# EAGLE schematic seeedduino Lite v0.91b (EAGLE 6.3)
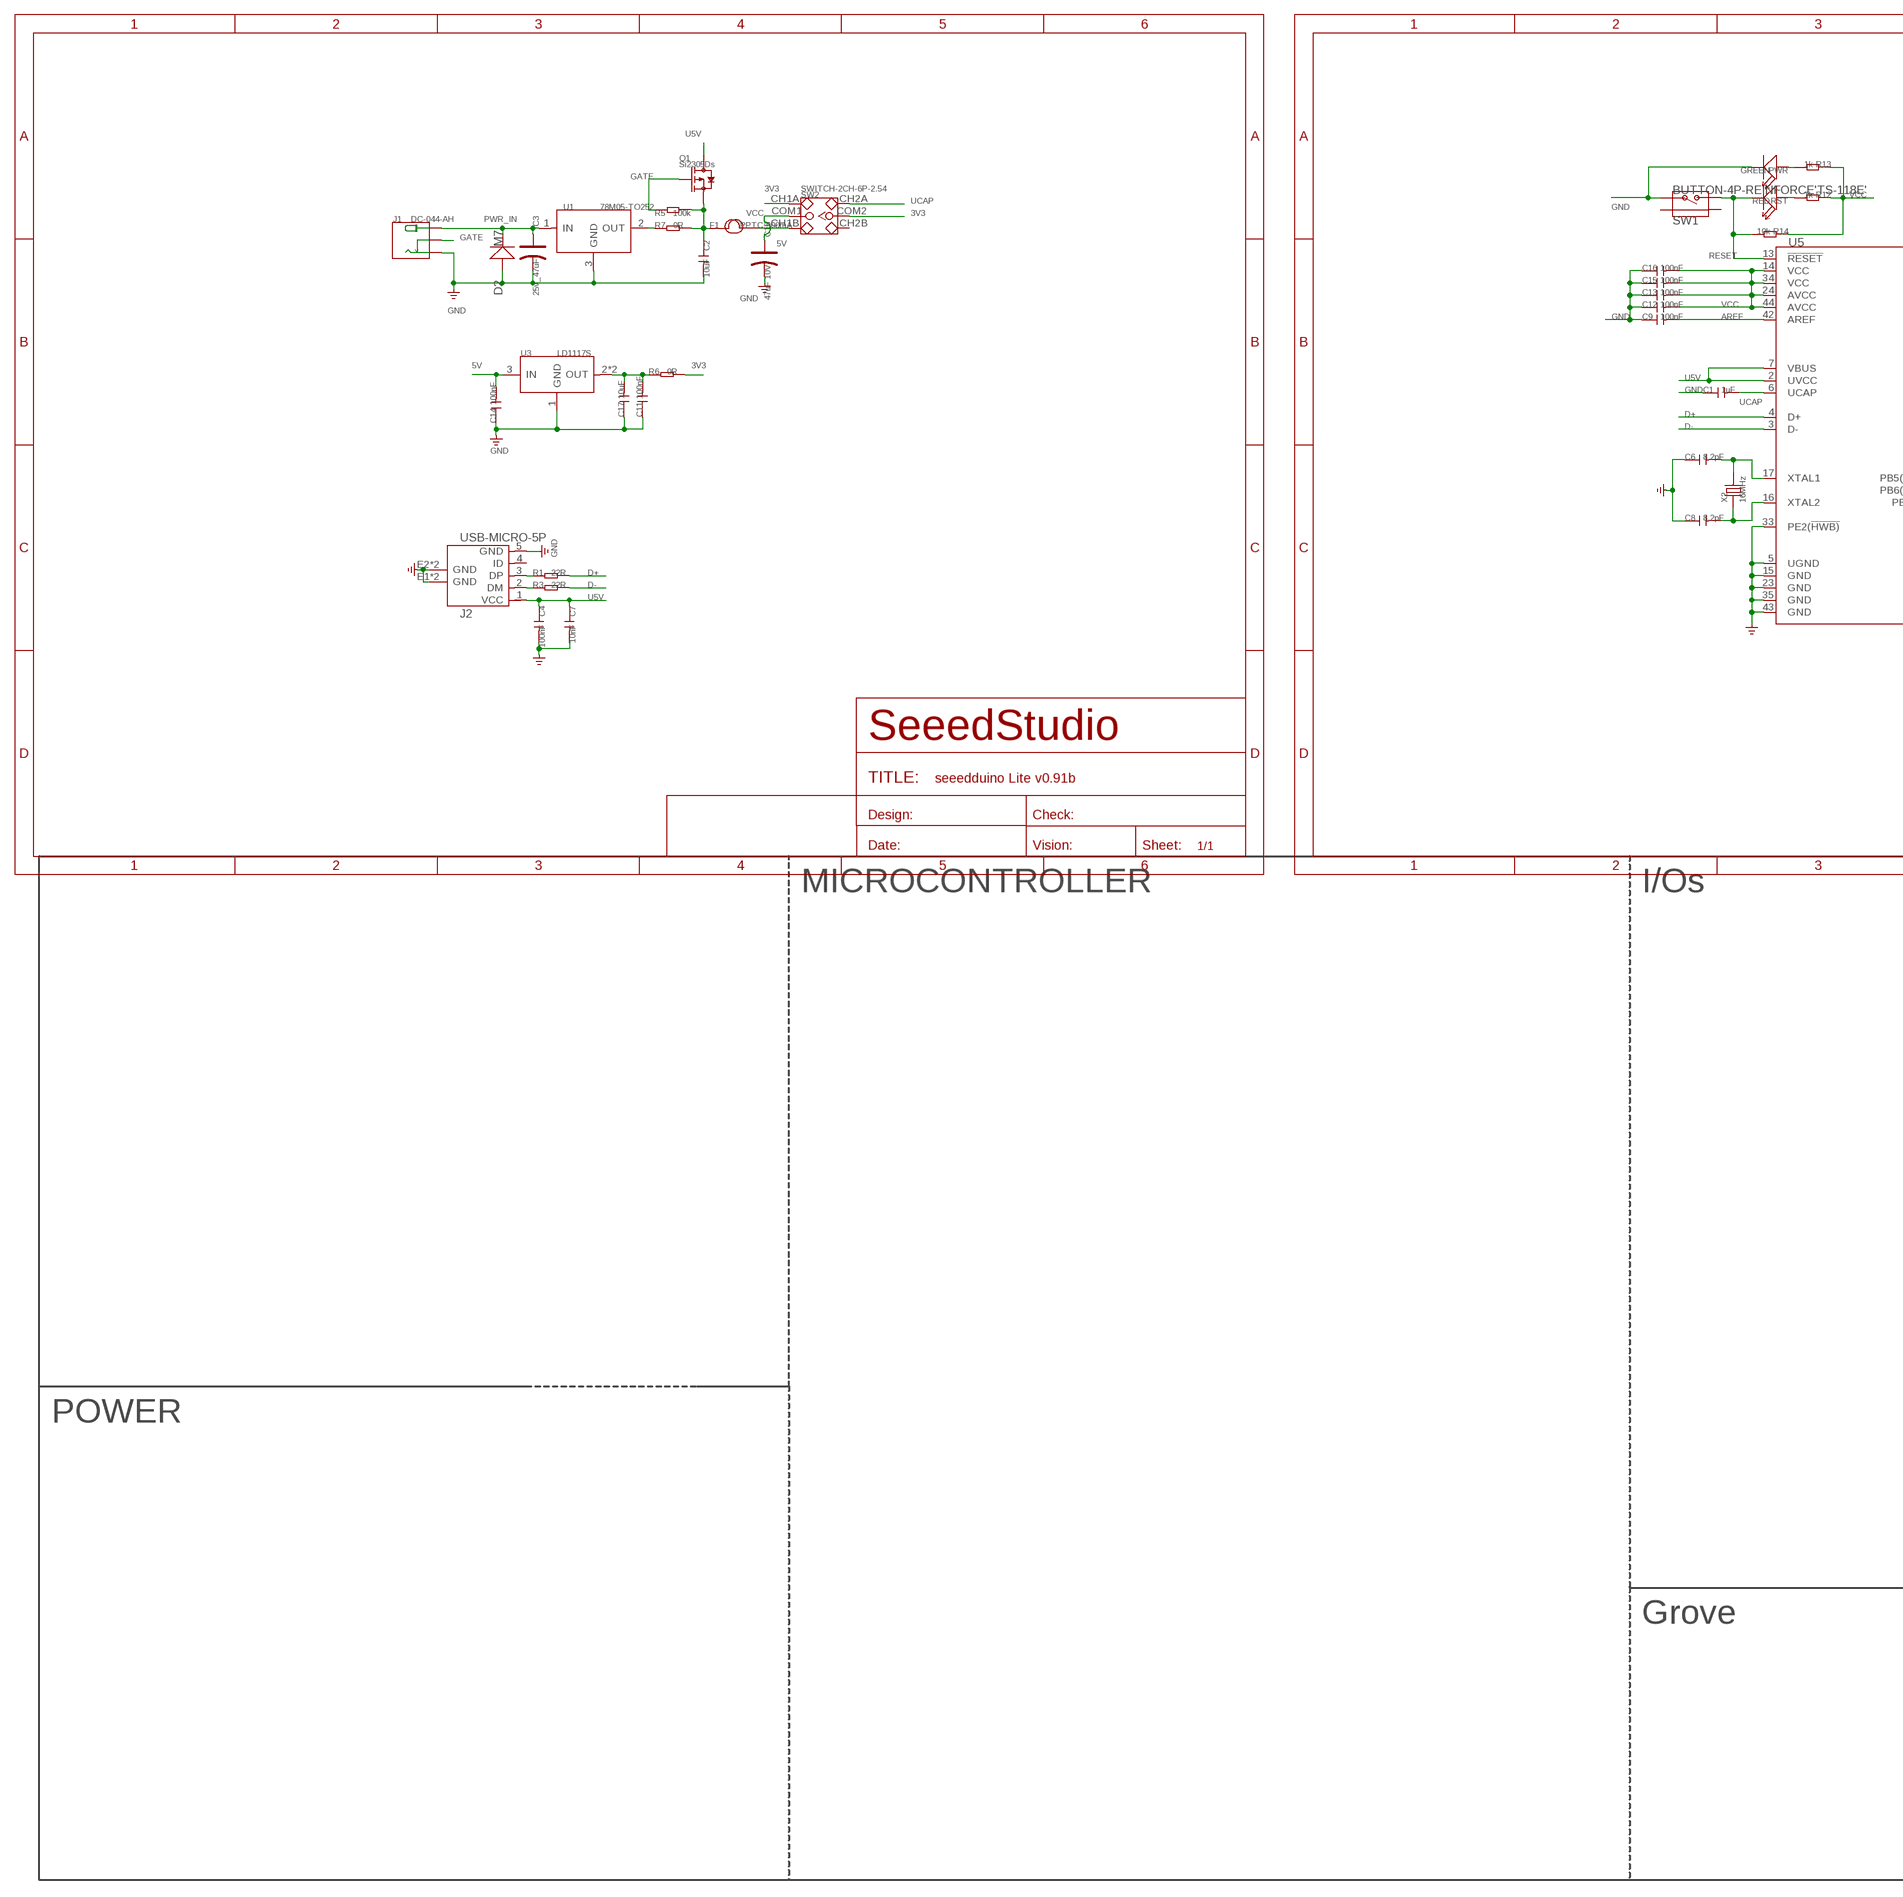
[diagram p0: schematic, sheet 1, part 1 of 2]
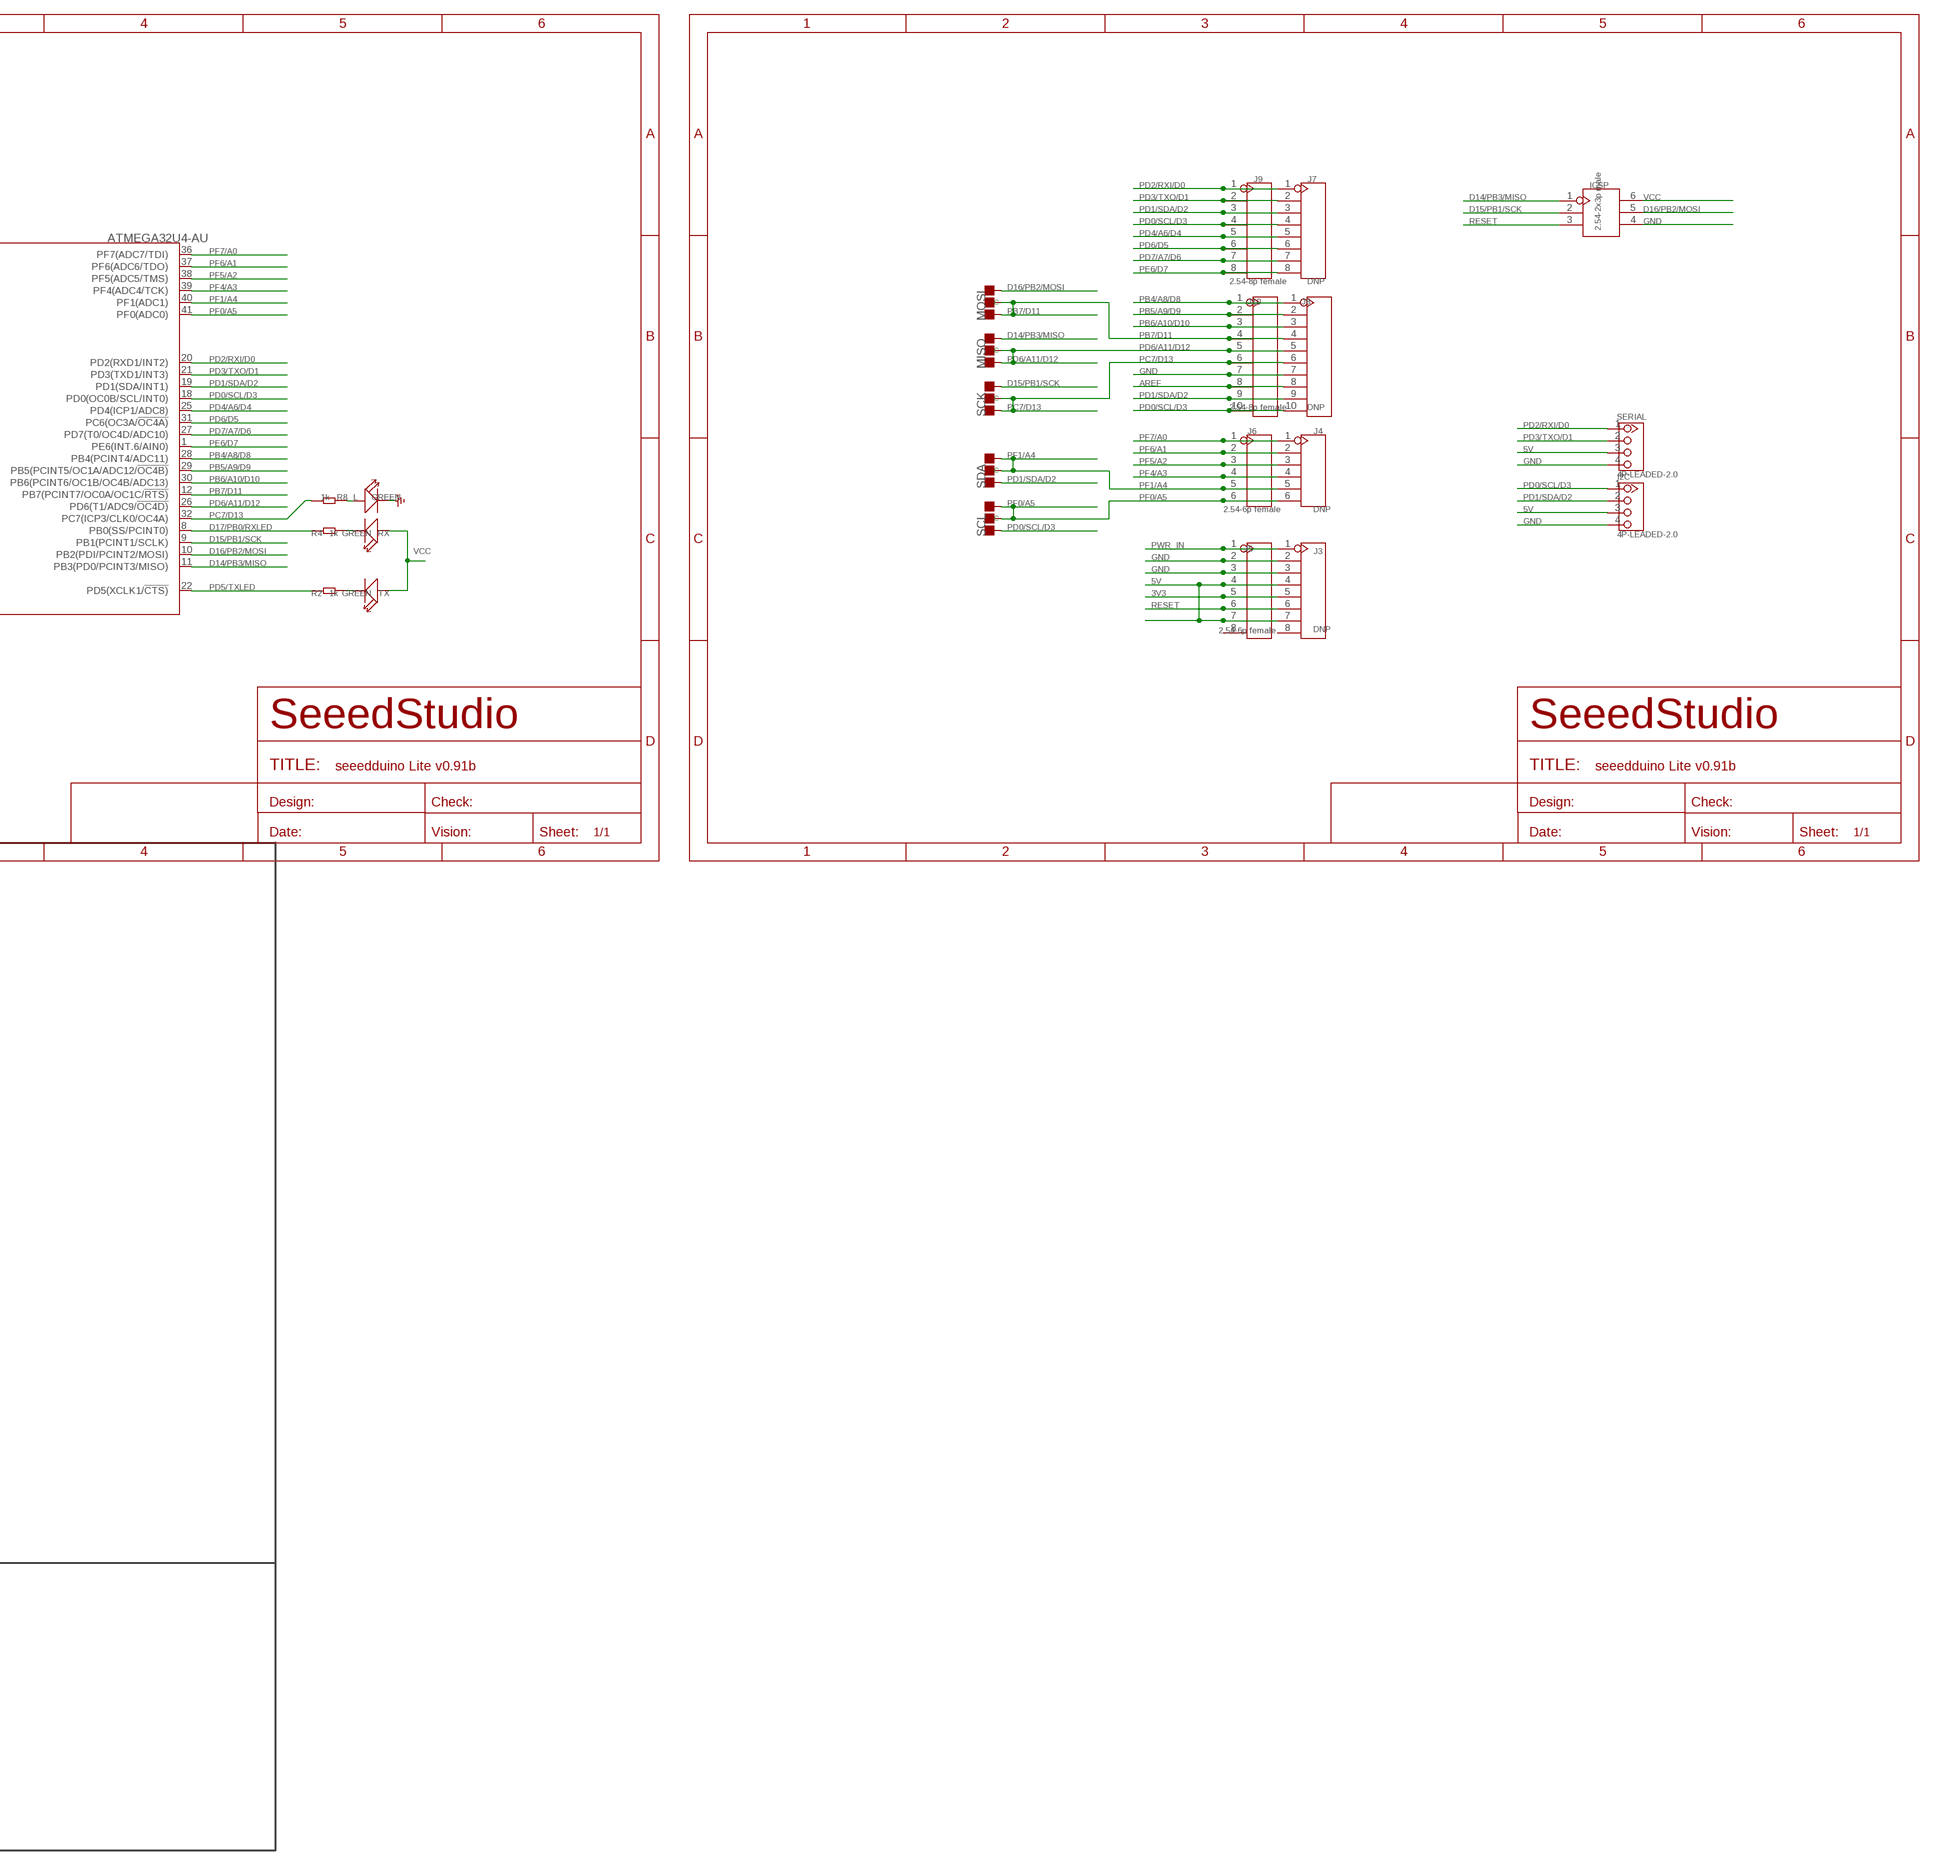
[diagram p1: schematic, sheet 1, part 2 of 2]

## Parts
C1  1uF  C-0805  [C0805]
C2  10uF  C-0805  [C0805]
C3  25v_47uF  CAP-ELECTRO-C  [ELECTRO-SMD-C-6MM]
C4  100nF  C-0603  [C0603]
C6  8.2pF  C-0603  [C0603]
C7  10nF  C-0603  [C0603]
C8  8.2pF  C-0603  [C0603]
C9  100nF  C-0603  [C0603]
C10  47uF 10V  CAP-AVX-B  [AVX-B]
C11  100nF  C-0603  [C0603]
C12  100nF  C-0603  [C0603]
C13  100nF  C-0603  [C0603]
C14  100nF  C-0603  [C0603]
C15  100nF  C-0603  [C0603]
C16  100nF  C-0603  [C0603]
C17  10uF  C-0805  [C0805]
D2  M7  D'SMA'  [D2010]
F1  PPTC-500mA  FUSE'1206'  [F1206]
I2C  4P-LEADED-2.0  TWIG-2.0-LEADED  [4P-LEADED-2.0]
ICSP  2.54-2x3p male  HEADER-2X3P-2.54  [2X3P-2.54]
J1  DC-044-AH  DC-044  [DC-404]
J2  USB-MICRO-5P  [MICRO-USB-5P]
J3  DNP  HEADER-8P-65/35MIL  [8P-2.54-65/35MIL]
J4  DNP  HEADER-6P-65/35MIL  [6P-2.54-65/35MIL]
J5  2.54-6p female  HEADER-8P-65/35MIL  [8P-2.54-65/35MIL]
J6  2.54-6p female  HEADER-6P-65/35MIL  [6P-2.54-65/35MIL]
J7  DNP  HEADER-8P-65/35MIL  [8P-2.54-65/35MIL]
J8  DNP  HEADER-10P-2.54  [10P-2.54]
J9  2.54-8p female  HEADER-8P-65/35MIL  [8P-2.54-65/35MIL]
J10  2.54-8p female  HEADER-10P-2.54  [10P-2.54]
L  GREEN  LED'0603'  [LED-0603]
MISO  DNP  PAD-JUMPER-3P-40*40  [3P-SMD-4.1X1.5]
MOSI  DNP  PAD-JUMPER-3P-40*40  [3P-SMD-4.1X1.5]
PWR  GREEN  LED'0603'  [LED-0603]
Q1  Si2305Ds  MOSFET-P'SI2323CDS/SI2305DS<BR>'  [SOT23]
R1  22R  R-0603  [R0603]
R2  1k  R-0603  [R0603]
R3  22R  R-0603  [R0603]
R4  1k  R-0603  [R0603]
R5  100k  R-0603  [R0603]
R6  0R  R-0603  [R0603]
R7  0R  R-0603  [R0603]
R8  1k  R-0603  [R0603]
R12  1k  R-0603  [R0603]
R13  1k  R-0603  [R0603]
R14  10k  R-0603  [R0603]
RST  RED  LED'0603'  [LED-0603]
RX  GREEN  LED'0603'  [LED-0603]
SCK  DNP  PAD-JUMPER-3P-40*40  [3P-SMD-4.1X1.5]
SCL  DNP  PAD-JUMPER-3P-40*40  [3P-SMD-4.1X1.5]
SDA  DNP  PAD-JUMPER-3P-40*40  [3P-SMD-4.1X1.5]
SERIAL  4P-LEADED-2.0  TWIG-2.0-LEADED  [4P-LEADED-2.0]
SW1  BUTTON-4P-REINFORCE'TS-118E'  [4P-SMD-7X3.5X3.5H]
SW2  SWITCH-2CH-6P-2.54  SWITCH-2CH-6P'MS-22D18'  [6P-2CH-2.5-9.1X3.5X3.2H]
TX  GREEN  LED'0603'  [LED-0603]
U1  78M05-TO252  [TO252]
U3  LD1117S  [SOT-223]
U5  ATMEGA32U4-AU  [TQFP44]
X2  16MHz  CRYSTAL'5032'  [2P-SMD-5X3.2]

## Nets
3V3: J3.5 J5.5 R6.2 SW2.CH1A SW2.COM2
5V [none3]: C14.2 F1.2 I2C.3 J3.4 J3.7 J5.4 J5.7 SERIAL.3 SW2.CH1B U3.3(IN)
AREF: C9.2 J8.8 J10.8 U5.42(AREF)
D14/PB3/MISO: ICSP.1 MISO.00(L) U5.11(PB3(PD0/PCINT3/MISO))
D15/PB1/SCK: ICSP.2 SCK.00(L) U5.9(PB1(PCINT1/SCLK))
D16/PB2/MOSI: ICSP.5 MOSI.00(L) U5.10(PB2(PDI/PCINT2/MOSI))
D17/PB0/RXLED: R4.1 U5.8(PB0(SS/PCINT0))
D+: R1.2 U5.4(D+)
D-: R3.2 U5.3(D-)
GATE: J1.CDN Q1.1(G) R5.1
GND [none1]: C1.1 C2.2 C3.- C4.2 C6.1 C7.2 C8.1 C9.1 C10.- C11.1 C12.1 C13.1 C14.1 C15.1 C16.1 C17.1 D2.+ I2C.4 ICSP.4 J1.- J2.5(GND) J2.E1(GND) J2.E2(GND) J2.P1(GND) J2.P2(GND) J3.2 J3.3 J5.2 J5.3 J8.7 J10.7 L.- PWR.- SERIAL.4 SW1.1 U1.3(GND) U3.1(GND) U5.5(UGND) U5.15(GND) U5.23(GND) U5.33(PE2(!HWB)) U5.35(GND) U5.43(GND)
N$1: C6.2 U5.17(XTAL1) X2.2
N$2: C8.2 U5.16(XTAL2) X2.1
N$3: C11.2 C17.2 R6.1 U3.2(OUT) U3.TER(OUT)
N$4: L.+ R8.1
N$5: R2.2 TX.-
N$6: J2.2(DM) R3.1
N$7: R4.2 RX.-
N$8: J2.3(DP) R1.1
N$9: C2.1 F1.1 Q1.2(S) R5.2 R7.2
N$10: PWR.+ R13.2
N$11: R7.1 U1.2(OUT)
N$17: R12.2 RST.+
PB4/A8/D8: J8.1 J10.1 U5.28(PB4(PCINT4/ADC11))
PB5/A9/D9: J8.2 J10.2 U5.29(PB5(PCINT5/OC1A/ADC12/!OC4B))
PB6/A10/D10: J8.3 J10.3 U5.30(PB6(PCINT6/OC1B/OC4B/ADC13))
PB7/D11: J8.4 J10.4 MOSI.11(R) MOSI.MM(C) U5.12(PB7(PCINT7/OC0A/OC1C/!RTS))
PC7/D13: J8.6 J10.6 R8.2 SCK.11(R) SCK.MM(C) U5.32(PC7(ICP3/CLK0/OC4A))
PD0/SCL/D3: I2C.1 J7.4 J8.10 J9.4 J10.10 SCL.11(R) U5.18(PD0(OC0B/SCL/INT0))
PD1/SDA/D2: I2C.2 J7.3 J8.9 J9.3 J10.9 SDA.11(R) U5.19(PD1(SDA/INT1))
PD2/RXI/D0: J7.1 J9.1 SERIAL.1 U5.20(PD2(RXD1/INT2))
PD3/TXO/D1: J7.2 J9.2 SERIAL.2 U5.21(PD3(TXD1/INT3))
PD4/A6/D4: J7.5 J9.5 U5.25(PD4(ICP1/ADC8))
PD5/TXLED: R2.1 U5.22(PD5(XCLK1/!CTS))
PD6/A11/D12: J8.5 J10.5 MISO.11(R) MISO.MM(C) U5.26(PD6(T1/ADC9/!OC4D))
PD6/D5: J7.6 J9.6 U5.31(PC6(OC3A/!OC4A))
PD7/A7/D6: J7.7 J9.7 U5.27(PD7(T0/OC4D/ADC10))
PE6/D7: J7.8 J9.8 U5.1(PE6(INT.6/AIN0))
PF0/A5: J4.6 J6.6 SCL.00(L) SCL.MM(C) U5.41(PF0(ADC0))
PF1/A4: J4.5 J6.5 SDA.00(L) SDA.MM(C) U5.40(PF1(ADC1))
PF4/A3: J4.4 J6.4 U5.39(PF4(ADC4/TCK))
PF5/A2: J4.3 J6.3 U5.38(PF5(ADC5/TMS))
PF6/A1: J4.2 J6.2 U5.37(PF6(ADC6/TDO))
PF7/A0: J4.1 J6.1 U5.36(PF7(ADC7/TDI))
PWR_IN: C3.+ D2.- J1.+ J3.1 J5.1 U1.1(IN)
RESET: ICSP.3 J3.6 J5.6 R14.2 RST.- SW1.2 U5.13(!RESET)
U5V: C4.1 C7.1 J2.1(VCC) Q1.3(D) U5.2(UVCC) U5.7(VBUS)
UCAP: C1.2 SW2.CH2A U5.6(UCAP)
VCC: C10.+ C12.2 C13.2 C15.2 C16.2 ICSP.6 R12.1 R13.1 R14.1 RX.+ SW2.COM1 TX.+ U5.14(VCC) U5.24(AVCC) U5.34(VCC) U5.44(AVCC)
Unconnected: J2.4(ID) J3.8 J5.8 SW1.S1 SW1.S2 SW2.CH2B

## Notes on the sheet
- MICROCONTROLLER | I/Os
- POWER
- Grove

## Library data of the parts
C1 C2 C4 C6-C9 C11-C17 = Discrete:C*: Ceramic Capacitors
C3 C10 = Discrete:CAP*: Electrolytic Capacitors,Tantalum Capacitors and Super Capacitors
D2 = Discrete:D*
F1 = Discrete:FUSE
I2C SERIAL = Connector:TWIG-2.0-LEADED
ICSP = Connector:HEADER-2X3P
J1 = For_Test_Albert:DC-044
J2 = Connector:USB-MICRO-5P
J3 J5 J7 J9 = Connector:HEADER-8P
J4 J6 = Connector:HEADER-6P
J8 J10 = Connector:HEADER-10P
L PWR RST RX TX = Discrete:LED*
MISO MOSI SCK SCL SDA = Discrete:PAD-JUMPER-3P; PARTNO: DNP
Q1 = Discrete:MOSFET-P
R1-R8 R12-R14 = Discrete:R*
SW1 = Discrete:BUTTON-4P-REINFORCE: TS-1188E http://www.best-dz.com/?thread-374-2.html
SW2 = Discrete:SWITCH-2CH-6P
U1 = IC:78M05: 0.5A Three Terminal Positive Voltage Regulators
U3 = IC:LD1117: Low Drop Fixed And Adjustable Positive Voltage Regulators http://www.datasheetcatalog.org/datasheet/SGSThomsonMicroelectronics/mXuqtqv.pdf
U5 = IC:ATMEGA32U4: 8-bit Microcontroller With 16/32K Bytes of ISP Flash and USB controller
X2 = Discrete:CRYSTAL*: CRYSTAL

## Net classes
0 default: width 0.152 mm, drill 0.305 mm, clearance 0.152 mm
3 none3: width 0.203 mm, drill 0.305 mm, clearance 0.203 mm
